{attribute 'c++_compatible'}
FUNCTION_BLOCK FB_Calculation EXTENDS TcBaseModuleRegistered IMPLEMENTS I_Calculation

VAR
END_VAR

{attribute 'c++_compatible'}
{attribute 'pack_mode' := '4'}
{attribute 'show'}
{attribute 'minimal_input_size' := '4'}
METHOD Addition : HRESULT
VAR_INPUT
	nIn1	: INT;
	nIn2	: INT;
	nRes	: REFERENCE TO INT;
END_VAR
nRes := nIn1 + nIn2;
END_METHOD

{attribute 'c++_compatible'}
{attribute 'pack_mode' := '4'}
{attribute 'show'}
{attribute 'minimal_input_size' := '4'}
METHOD Subtraction : HRESULT
VAR_INPUT
	nIn1	: INT;
	nIn2	: INT;
	nRes	: REFERENCE TO INT;
END_VAR
nRes := nIn1 - nIn2;
END_METHOD

{attribute 'c++_compatible'}
{attribute 'pack_mode' := '4'}
{attribute 'show'}
{attribute 'minimal_input_size' := '4'}
METHOD TcQueryInterface : HRESULT
VAR_INPUT
	iid	: REFERENCE TO IID;
	pipItf	: POINTER TO PVOID;
END_VAR

VAR
	ipCalc : I_Calculation;
END_VAR
IF GuidsEqual(ADR(iid), ADR(TC_GLOBAL_IID_LIST.IID_I_Calculation)) THEN
	ipCalc := THIS^; 
	pipItf^ := ITCUNKNOWN_TO_PVOID(ipCalc);
	TcAddRef();
	TcQueryInterface := S_OK;
ELSE
	TcQueryInterface := SUPER^.TcQueryInterface(iid, pipItf);
END_IF
END_METHOD

END_FUNCTION_BLOCK
